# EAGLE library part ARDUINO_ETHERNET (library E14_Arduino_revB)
Device for representing an Arduino Ethernet board with a footprint in an EAGLE design. Created by Dave Young for Element14. More EAGLE documentation at: http://www.element14.com/community/community/knode/cadsoft_eagle
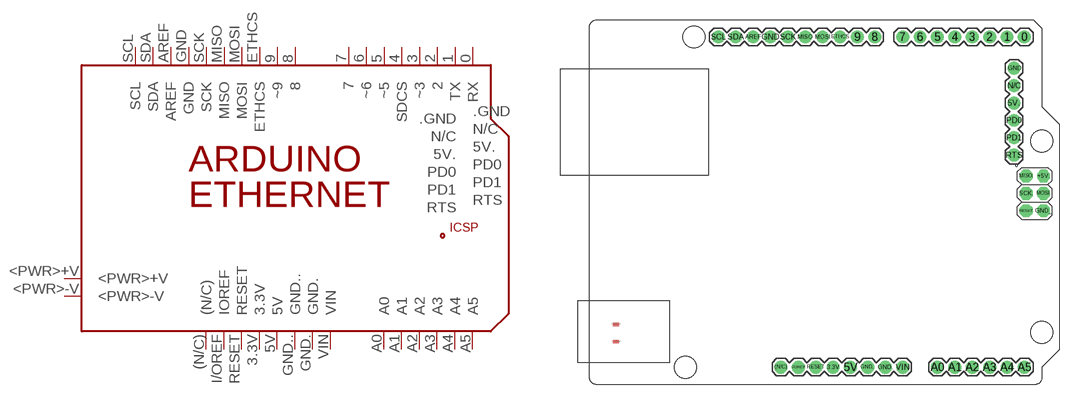
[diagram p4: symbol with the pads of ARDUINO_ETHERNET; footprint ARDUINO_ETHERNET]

Designator prefix PCB

## ARDUINO_ETHERNET  [ARDUINO_ETHERNET]
0  RX
1  TX
2  2
3  ~3
3.3V  3.3V
4  SDCS
5  ~5
5V  5V
5V.  5V.
6  ~6
7  7
8  8
9  ~9
(N/C)  (N/C)
+5V.  +5V.
.GND  .GND
<PWR>+V  <PWR>+V
<PWR>-V  <PWR>-V
A0  A0
A1  A1
A2  A2
A3  A3
A4  A4
A5  A5
AREF  AREF
ETHCS  ETHCS
GND  GND
GND.  GND.
GND..  GND..
GND_  GND_
I/OREF  IOREF
MISO  MISO
MISO.  MISO.
MOSI  MOSI
MOSI.  MOSI.
N/C  N/C
PD0  PD0
PD1  PD1
RESET  RESET
RESET.  RESET.
RTS  RTS
SCK  SCK
SCK.  SCK.
SCL  SCL
SDA  SDA
VIN  VIN

## Footprint ARDUINO_ETHERNET (pad centres in mm)
Footprint for representing an Arduino Ethernet board in an EAGLE schematic. Created by Dave Young for Element14. More EAGLE documentation at: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
drill 1.016 pad 1.88: 0 63.5,50.8; 1 60.96,50.8; 2 58.42,50.8; 3 55.88,50.8; 3.3V 35.56,2.54; 4 53.34,50.8; 5 50.8,50.8; 5V 38.1,2.54; 5V. 61.976,41.148; 6 48.26,50.8; 7 45.72,50.8; 8 41.656,50.8; 9 39.116,50.8; (N/C) 27.94,2.54; .GND 61.976,46.228; A0 50.8,2.54; A1 53.34,2.54; A2 55.88,2.54; A3 58.42,2.54; A4 60.96,2.54; A5 63.5,2.54; AREF 23.876,50.8; ETHCS 36.576,50.8; GND 26.416,50.8; GND. 43.18,2.54; GND.. 40.64,2.54; I/OREF 30.48,2.54; MISO 31.496,50.8; MOSI 34.036,50.8; N/C 61.976,43.688; PD0 61.976,38.608; PD1 61.976,36.068; RESET 33.02,2.54; RTS 61.976,33.528; SCK 28.956,50.8; SCL 18.796,50.8; SDA 21.336,50.8; VIN 45.72,2.54
drill 1.016 pad 1.88 octagon: +5V. 66.294,30.48; GND_ 66.294,25.4; MISO. 63.754,30.48; MOSI. 66.294,27.94; RESET. 63.754,25.4; SCK. 63.754,27.94
smd 1.016 x 0.508: <PWR>+V 3.861,8.814; <PWR>-V 3.861,6.274
hole 3.2 at 66.04,7.62
hole 3.2 at 66.04,35.56
hole 3.2 at 15.24,50.8
hole 3.2 at 13.97,2.54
